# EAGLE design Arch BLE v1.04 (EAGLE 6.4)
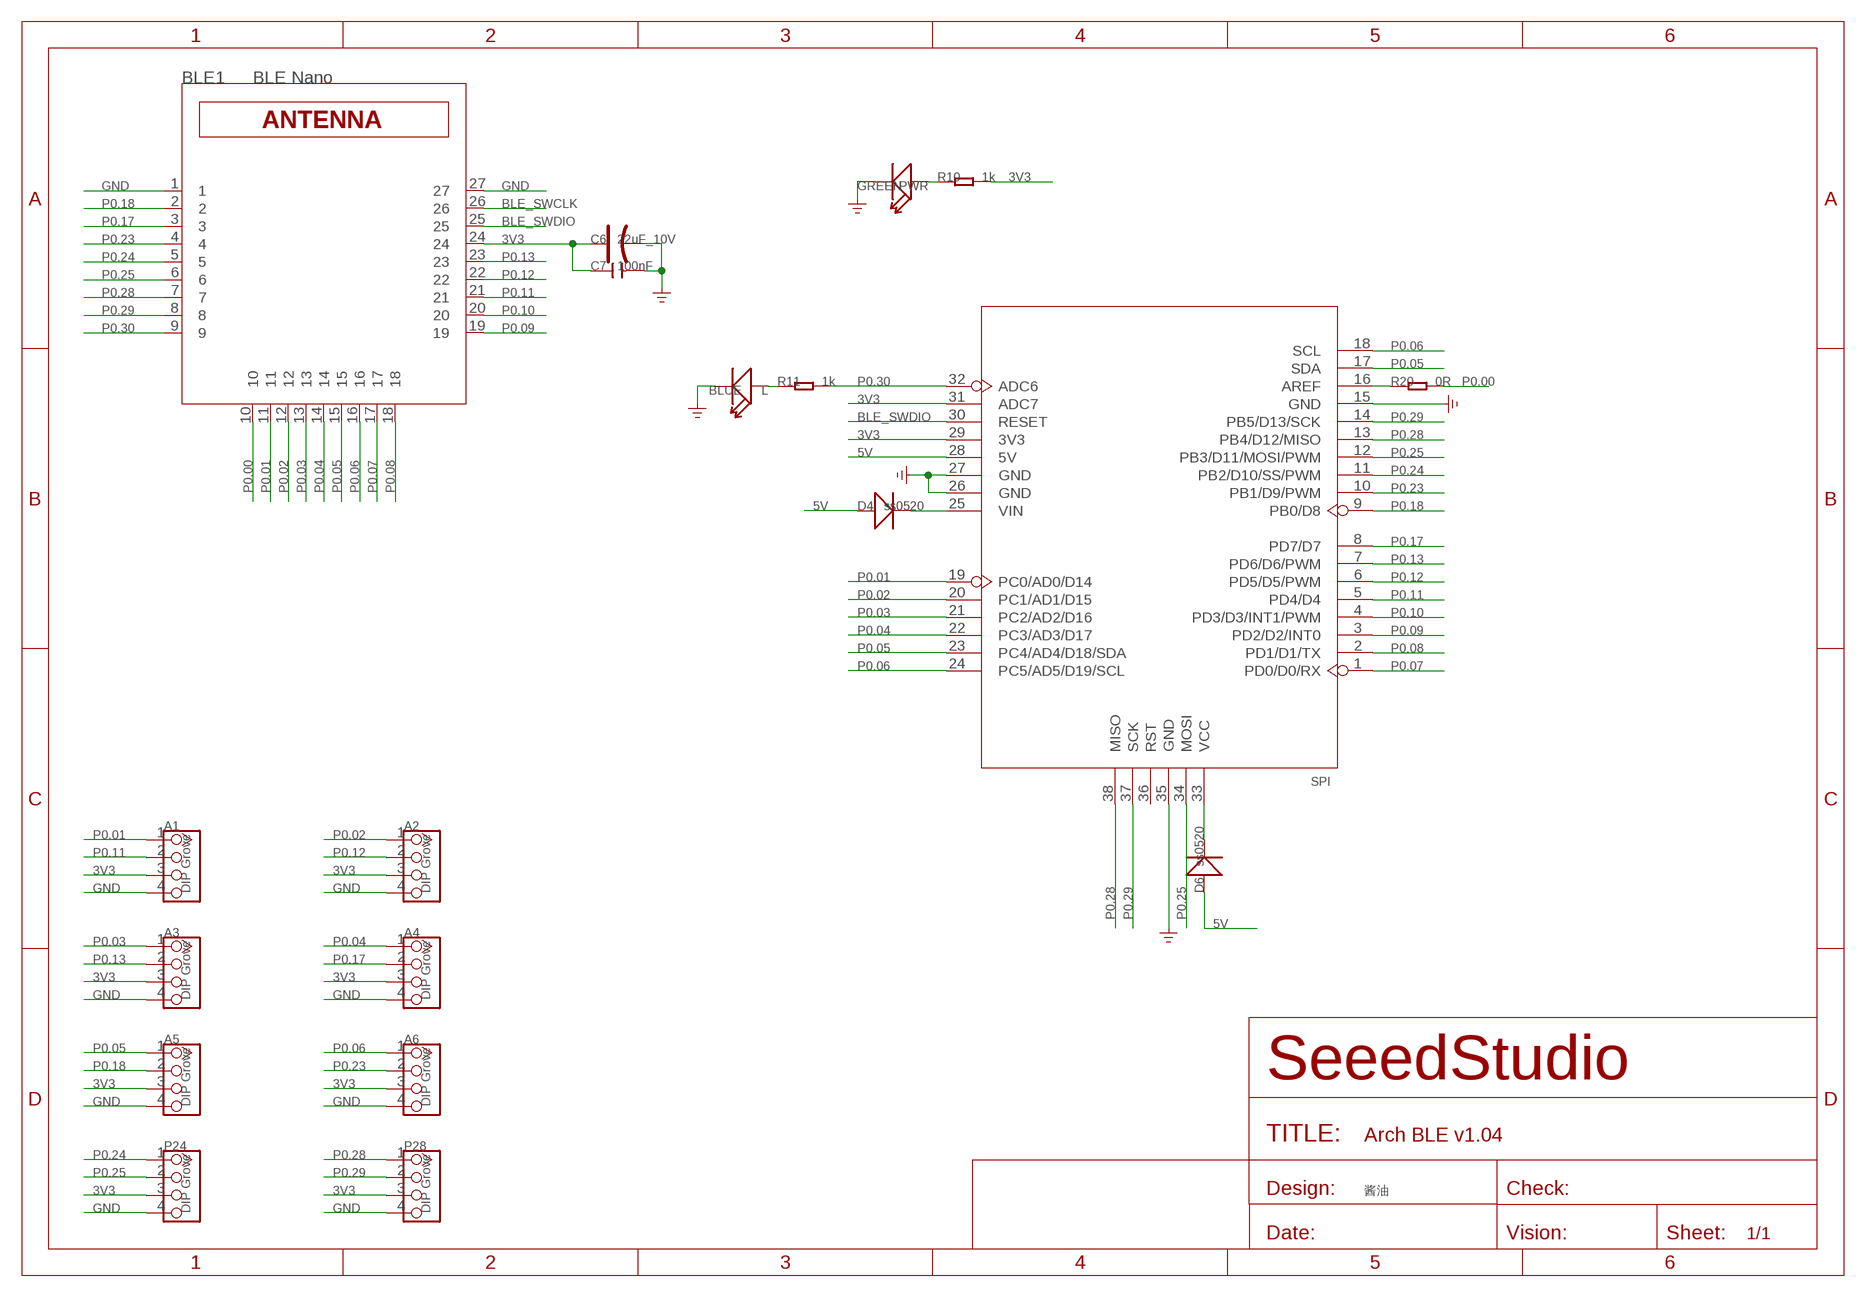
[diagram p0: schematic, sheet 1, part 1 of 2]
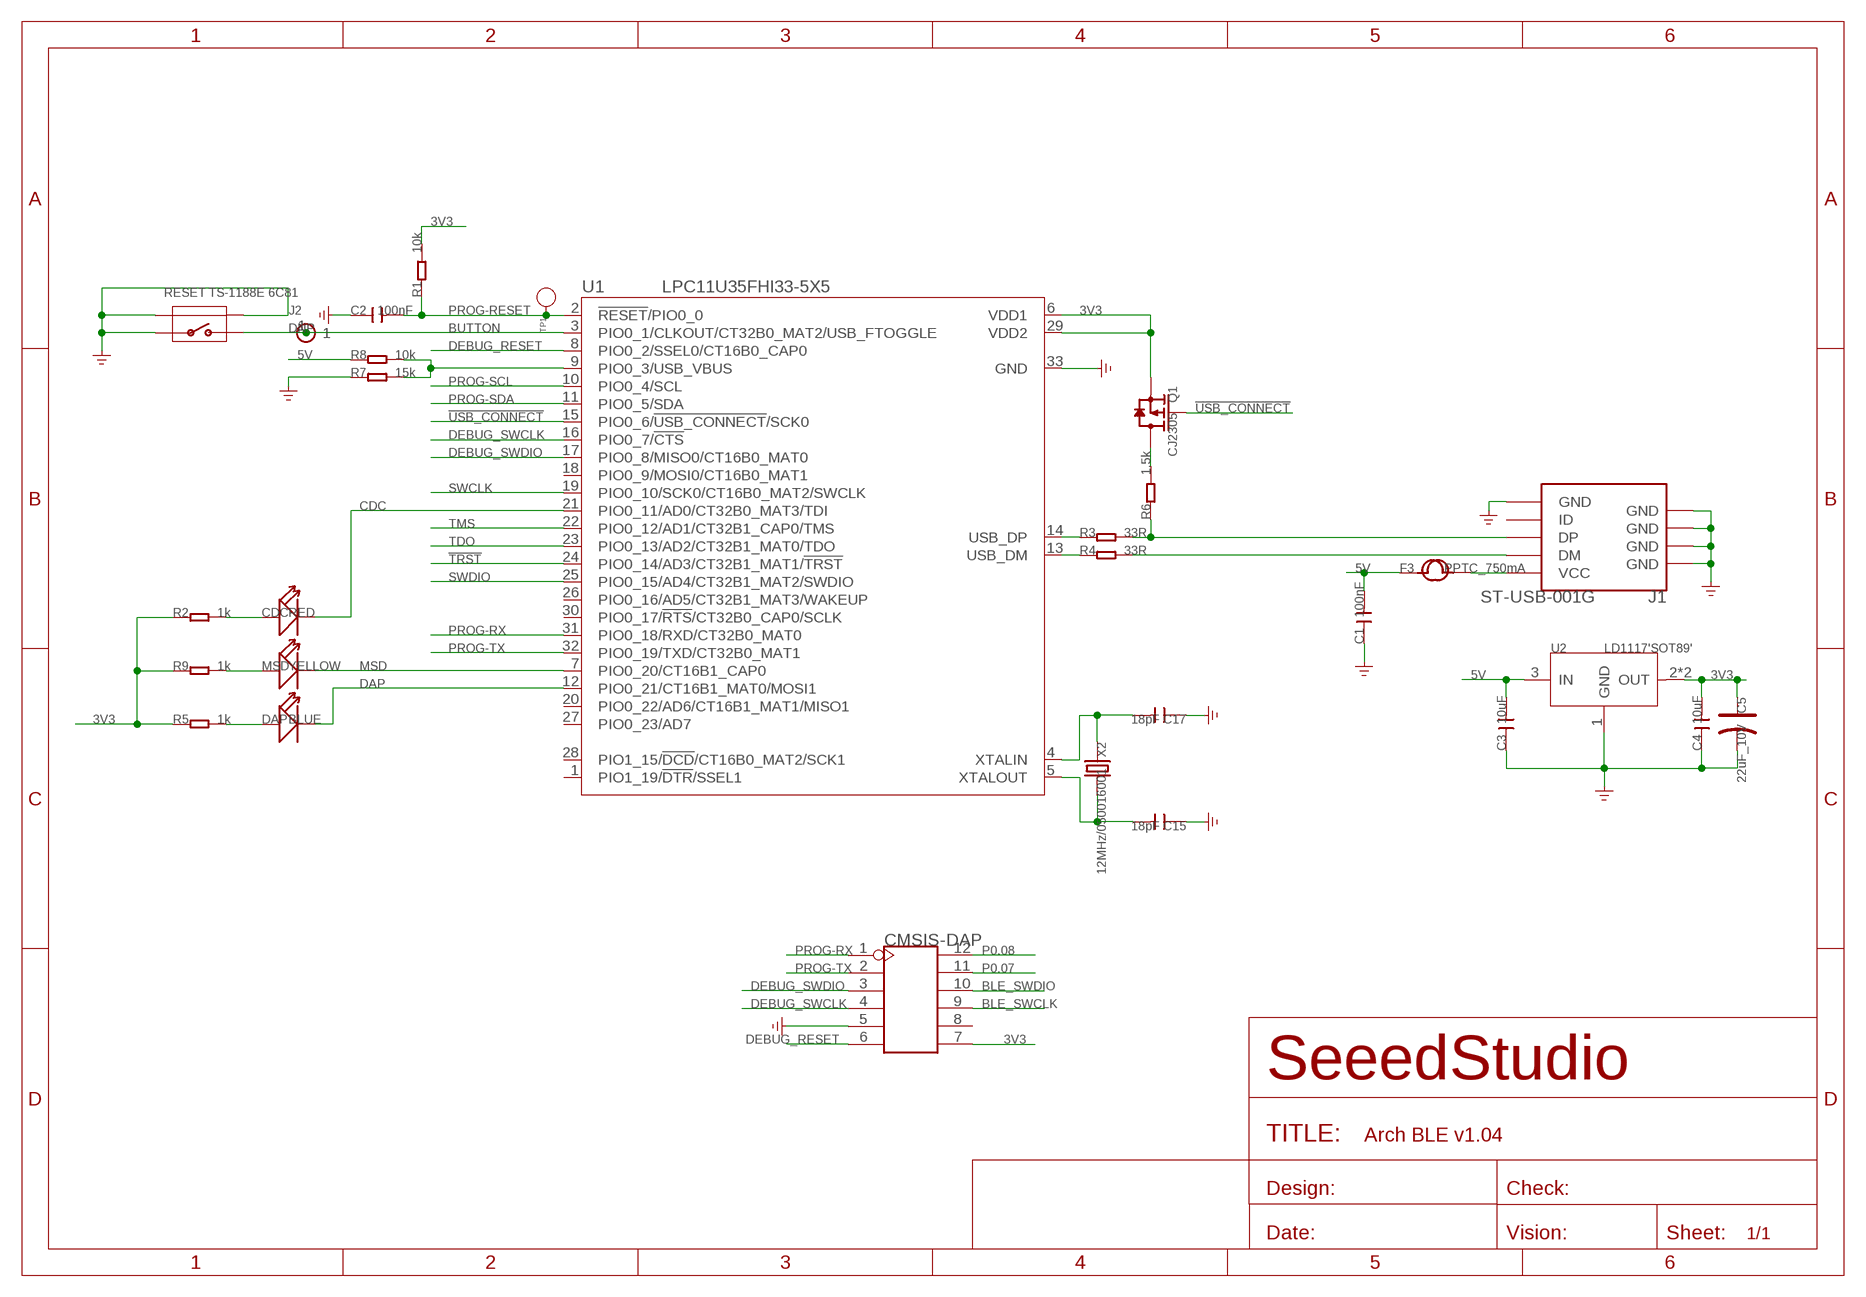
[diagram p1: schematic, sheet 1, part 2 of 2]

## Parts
A1  DIP Grove  TWIG-4P-2.0-2.0  [4P-2.0]
A2  DIP Grove  TWIG-4P-2.0-2.0  [4P-2.0]
A3  DIP Grove  TWIG-4P-2.0-2.0  [4P-2.0]
A4  DIP Grove  TWIG-4P-2.0-2.0  [4P-2.0]
A5  DIP Grove  TWIG-4P-2.0-2.0  [4P-2.0]
A6  DIP Grove  TWIG-4P-2.0-2.0  [4P-2.0]
BLE1  BLE Nano  SEEED_BLE_MODULE_001'PAD'  [SEEED_BLE_MODULE_PAD]
C1  100nF  C-0603  [C0603]
C2  100nF  C-0603  [C0603]
C3  10uF  C-0805  [C0805]
C4  10uF  C-0805  [C0805]
C5  22uF_10V  CAP-AVX-A  [AVX-A]
C6  22uF_10V  CAP-AVX-A  [AVX-A]
C7  100nF  C-0603  [C0603]
C15  18pF  C-0603  [C0603]
C17  18pF  C-0603  [C0603]
CDC  RED  LED'0603'  [LED-0603]
CMSIS-DAP  HEADER-2X6P-2.54  [2X6P-2.54]
D4  ss0520  D'1206'  [SOD123]
D6  ss0520  D'1206'  [SOD123]
DAP  BLUE  LED'0603'  [LED-0603]
F3  PPTC_750mA  FUSE'1206'  [F1206]
J1  ST-USB-001G  USB-MINIUSB-5P-MICRO  [MICRO-USB]
J2  DNP  HEADER-1P-35  [1P-65/35MIL]
L  BLUE  LED'0603'  [LED-0603]
MSD  YELLOW  LED'0603'  [LED-0603]
P24  DIP Grove  TWIG-4P-2.0-2.0  [4P-2.0]
P28  DIP Grove  TWIG-4P-2.0-2.0  [4P-2.0]
PWR  GREEN  LED'0603'  [LED-0603]
Q1  CJ2305  MOSFET-P'SI2323CDS/SI2305DS<BR>'  [SOT23]
R1  10k  R-0603  [R0603]
R2  1k  R-0603  [R0603]
R3  33R  R-0603  [R0603]
R4  33R  R-0603  [R0603]
R5  1k  R-0603  [R0603]
R6  1.5k  R-0603  [R0603]
R7  15k  R-0603  [R0603]
R8  10k  R-0603  [R0603]
R9  1k  R-0603  [R0603]
R10  1k  R-0603  [R0603]
R11  1k  R-0603  [R0603]
R20  0R  R-0603  [R0603]
RESET  TS-1188E 6C81  BUTTON-4P-REINFORCE'TS-1188E'  [4P-SMD-7X3.5X3.5H]
TP1  PAD-TEST-POINT'4545'  [TP_4545]
U1  LPC11U35FHI33-5X5  [HVQFN33]
U2  LD1117'SOT89'  [SOT89]
U5  ARDUINO-38P'WITH/O-SILK'  [ARDUINO-38P]
X2  12MHz/050016001  CRYSTAL'5032'  [2P-SMD-5X3.2]

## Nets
3V3: A1.3 A2.3 A3.3 A4.3 A5.3 A6.3 BLE1.24 C4.2 C5.+ C6.+ C7.1 CMSIS-DAP.7 P24.3 P28.3 Q1.2(S) R1.2 R2.1 R5.1 R9.1 R10.2 U1.6(VDD1) U1.29(VDD2) U2.2(OUT) U2.4(OUT) U5.29(3V3) U5.31(ADC7)
5V: C1.2 C3.2 D4.+ D6.+ F3.1 R8.1 U2.3(IN) U5.28(5V)
!TRST: U1.24(PIO0_14/AD3/CT32B1_MAT1/!TRST!)
!USB_CONNECT: Q1.1(G) U1.15(PIO0_6/!USB_CONNECT!/SCK0)
BLE_SWCLK: BLE1.26 CMSIS-DAP.9
BLE_SWDIO: BLE1.25 CMSIS-DAP.10 U5.30(RESET)
BUTTON: J2.1 RESET.2 U1.3(PIO0_1/CLKOUT/CT32B0_MAT2/USB_FTOGGLE)
CDC: CDC.- U1.21(PIO0_11/AD0/CT32B0_MAT3/TDI)
DAP: DAP.- U1.12(PIO0_21/CT16B1_MAT0/MOSI1)
DEBUG_RESET: CMSIS-DAP.6 U1.8(PIO0_2/SSEL0/CT16B0_CAP0)
DEBUG_SWCLK: CMSIS-DAP.4 U1.16(PIO0_7/!CTS!)
DEBUG_SWDIO: CMSIS-DAP.3 U1.17(PIO0_8/MISO0/CT16B0_MAT0)
GND: A1.4 A2.4 A3.4 A4.4 A5.4 A6.4 BLE1.1 BLE1.27 C1.1 C2.1 C3.1 C4.1 C5.- C6.- C7.2 C15.1 C17.1 CMSIS-DAP.5 J1.5(GND) J1.S1(GND) J1.S2(GND) J1.S3(GND) J1.S4(GND) J1.S5(GND) J1.S6(GND) L.- P24.4 P28.4 PWR.- R7.1 RESET.1 RESET.S1 RESET.S2 U1.33(GND) U2.1(GND) U5.15(GND) U5.26(GND) U5.27(GND) U5.35(GND)
MSD: MSD.- U1.7(PIO0_20/CT16B1_CAP0)
N$1: R3.1 U1.14(USB_DP)
N$2: PWR.+ R10.1
N$3: F3.2 J1.1(VCC)
N$4: CDC.+ R2.2
N$5: DAP.+ R5.2
N$6: MSD.+ R9.2
N$8: R20.1 U5.16(AREF)
N$11: L.+ R11.1
N$12: D4.- U5.25(VIN)
N$14: D6.- U5.33(VCC)
N$23: R4.1 U1.13(USB_DM)
N$32: J1.3(DP) R3.2 R6.1
N$34: C15.2 U1.5(XTALOUT) X2.2
N$37: C17.2 U1.4(XTALIN) X2.1
N$38: J1.2(DM) R4.2
N$39: Q1.3(D) R6.2
N$41: R7.2 R8.2 U1.9(PIO0_3/USB_VBUS)
P0.00: BLE1.10 R20.2
P0.01: A1.1 BLE1.11 U5.19(PC0/AD0/D14)
P0.02: A2.1 BLE1.12 U5.20(PC1/AD1/D15)
P0.03: A3.1 BLE1.13 U5.21(PC2/AD2/D16)
P0.04: A4.1 BLE1.14 U5.22(PC3/AD3/D17)
P0.05: A5.1 BLE1.15 U5.17(SDA) U5.23(PC4/AD4/D18/SDA)
P0.06: A6.1 BLE1.16 U5.18(SCL) U5.24(PC5/AD5/D19/SCL)
P0.07: BLE1.17 CMSIS-DAP.11 U5.1(PD0/D0/RX)
P0.08: BLE1.18 CMSIS-DAP.12 U5.2(PD1/D1/TX)
P0.09: BLE1.19 U5.3(PD2/D2/INT0)
P0.10: BLE1.20 U5.4(PD3/D3/INT1/PWM)
P0.11: A1.2 BLE1.21 U5.5(PD4/D4)
P0.12: A2.2 BLE1.22 U5.6(PD5/D5/PWM)
P0.13: A3.2 BLE1.23 U5.7(PD6/D6/PWM)
P0.17: A4.2 BLE1.3 U5.8(PD7/D7)
P0.18: A5.2 BLE1.2 U5.9(PB0/D8)
P0.23: A6.2 BLE1.4 U5.10(PB1/D9/PWM)
P0.24: BLE1.5 P24.1 U5.11(PB2/D10/SS/PWM)
P0.25: BLE1.6 P24.2 U5.12(PB3/D11/MOSI/PWM) U5.34(MOSI)
P0.28: BLE1.7 P28.1 U5.13(PB4/D12/MISO) U5.38(MISO)
P0.29: BLE1.8 P28.2 U5.14(PB5/D13/SCK) U5.37(SCK)
P0.30: BLE1.9 R11.2 U5.32(ADC6)
PROG-RESET: C2.2 R1.1 TP1.T U1.2(!RESET!/PIO0_0)
PROG-RX: CMSIS-DAP.1 U1.31(PIO0_18/RXD/CT32B0_MAT0)
PROG-SCL: U1.10(PIO0_4/SCL)
PROG-SDA: U1.11(PIO0_5/SDA)
PROG-TX: CMSIS-DAP.2 U1.32(PIO0_19/TXD/CT32B0_MAT1)
SWCLK: U1.19(PIO0_10/SCK0/CT16B0_MAT2/SWCLK)
SWDIO: U1.25(PIO0_15/AD4/CT32B1_MAT2/SWDIO)
TDO: U1.23(PIO0_13/AD2/CT32B1_MAT0/TDO)
TMS: U1.22(PIO0_12/AD1/CT32B1_CAP0/TMS)
Unconnected: CMSIS-DAP.8 J1.4(ID) U1.1(PIO1_19/!DTR!/SSEL1) U1.18(PIO0_9/MOSI0/CT16B0_MAT1) U1.20(PIO0_22/AD6/CT16B1_MAT1/MISO1) U1.26(PIO0_16/AD5/CT32B1_MAT3/WAKEUP) U1.27(PIO0_23/AD7) U1.28(PIO1_15/!DCD!/CT16B0_MAT2/SCK1) U1.30(PIO0_17/!RTS!/CT32B0_CAP0/SCLK) U5.36(RST)

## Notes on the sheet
- SPI
- 酱油

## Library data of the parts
A1-A6 P24 P28 = Connector:TWIG-4P-2.0
BLE1 = AMLib:SEEED_BLE_MODULE_001
C1-C4 C7 C15 C17 = Discrete:C*: Ceramic Capacitors
C5 C6 = Discrete:CAP*: Electrolytic Capacitors,Tantalum Capacitors and Super Capacitors
CDC DAP L MSD PWR = Discrete:LED*
CMSIS-DAP = Connector:HEADER-2X6P
D4 D6 = Discrete:D*
F3 = Discrete:FUSE
J1 = Connector :USB-MINIUSB-5P
J2 = Connector :HEADER-1P
Q1 = Discrete:MOSFET-P
R1-R11 R20 = Discrete:R*
RESET = Discrete:BUTTON-4P-REINFORCE: TS-1188E http://www.best-dz.com/?thread-374-2.html
TP1 = Discrete:PAD-TEST-POINT; PARTNO: DNP
U1 = AMLib:LPC11U35FHI33
U2 = IC:LD1117: Low Drop Fixed And Adjustable Positive Voltage Regulators http://www.datasheetcatalog.org/datasheet/SGSThomsonMicroelectronics/mXuqtqv.pdf
U5 = moudle:ARDUINO-38P
X2 = Discrete:CRYSTAL*: CRYSTAL

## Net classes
0 default: width 0.102 mm, drill 0.203 mm, clearance 0.102 mm

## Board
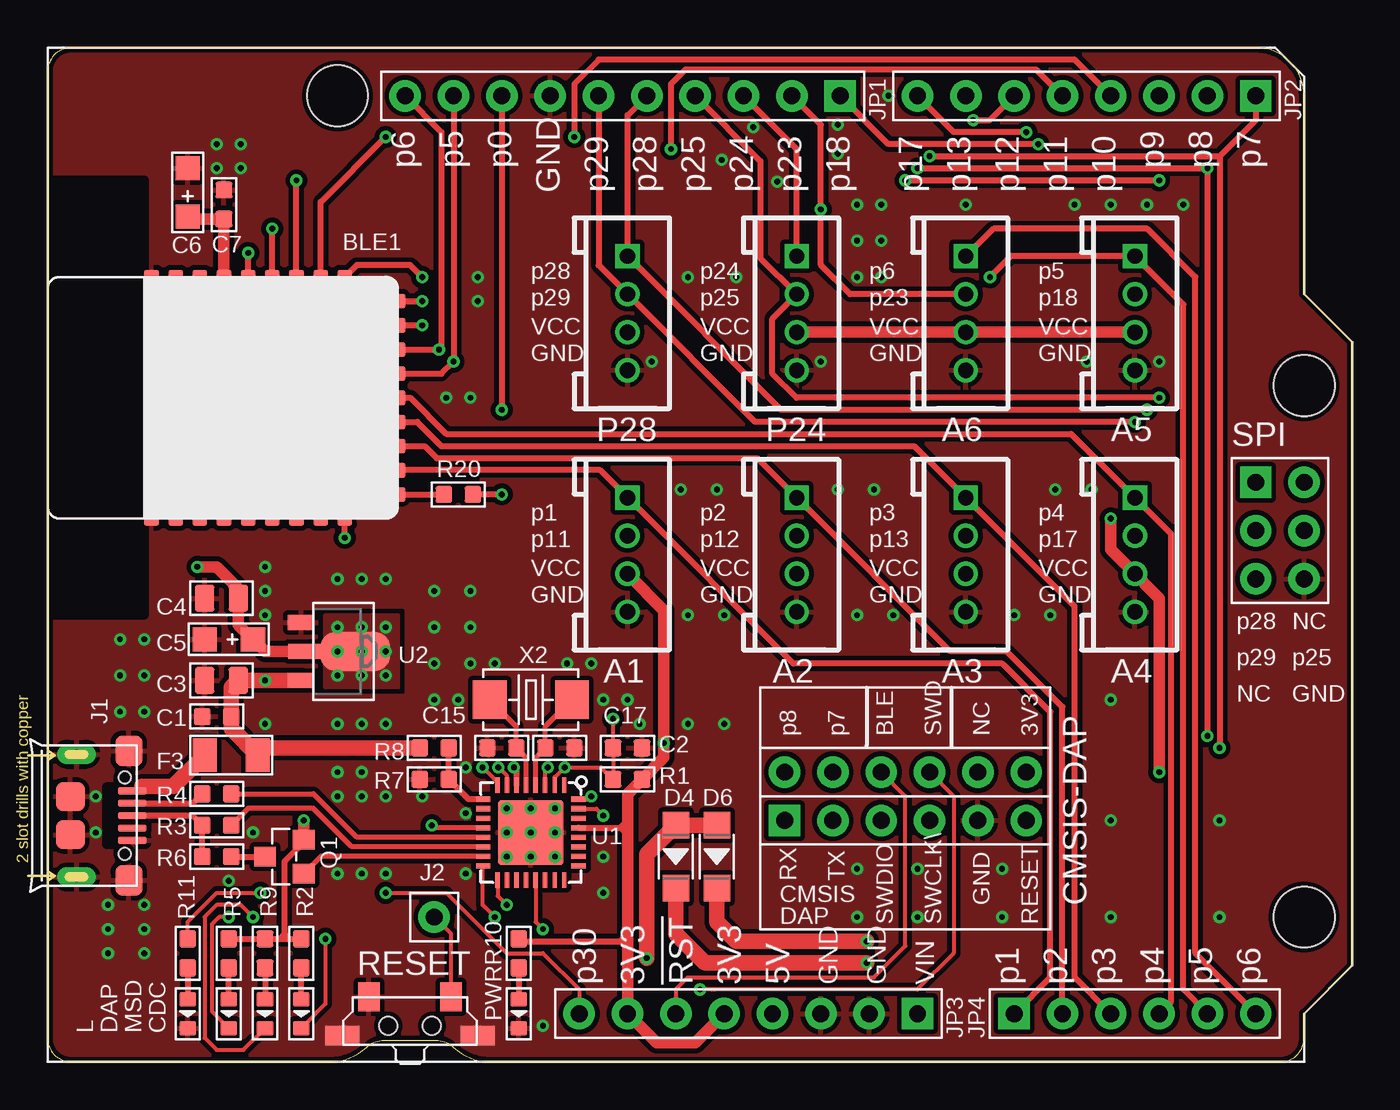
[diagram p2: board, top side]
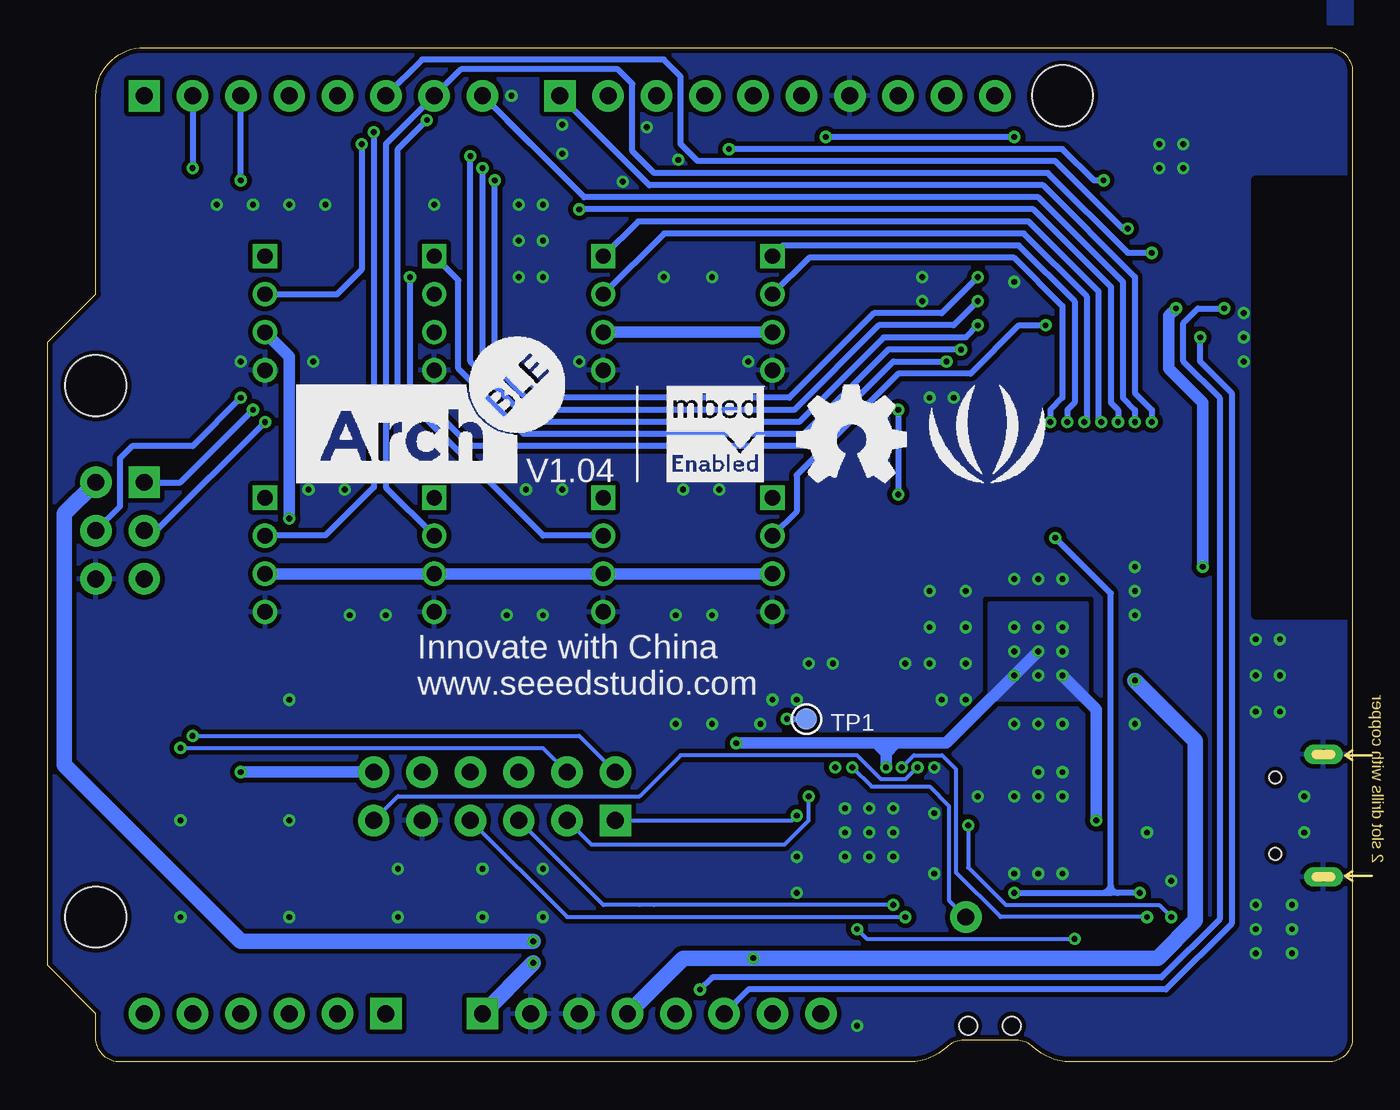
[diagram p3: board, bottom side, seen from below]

Size 68.58 x 53.34 mm. Coordinates in mm from the lower left corner, seen from the top.
Outline: 66.04,40.39 66.04,50.8 arc90 63.5,53.34 1.27,53.34 arc90 0,52.07 0,1.27 arc90 1.27,0 14.61,0 arc45 16.77,0.77 arc-45 17.67,1.14 20.43,1.14 arc-45 21.33,0.77 arc45 23.5,0 64.77,0 arc90 66.04,1.27 66.04,2.54 68.58,5.08 68.58,37.85 66.04,40.39
Copper layers (1*16): Top 0.035mm / dielectric 1.5mm / Bottom 0.035mm
Design rules "default *": minimum track width 6mil, minimum drill 12mil, track to track 6mil, track to pad 6mil, pad to pad 6mil, via to via 6mil, smd to smd 0mil, copper to edge 6mil, drill to drill 8mil, minimum pad ring 6mil, minimum via ring 6mil, stop-mask expansion 4mil, vias tented up to drill 25mil, thermal gap 10mil
tRestrict: area -0.6,23.5 to 5.1,46.4
bRestrict: area -0.6,23.5 to 5.1,46.4

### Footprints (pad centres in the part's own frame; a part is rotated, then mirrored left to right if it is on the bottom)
4P-2.0 = drill 0.8 pad 1.27 square: 1 -3,0 | drill 0.8 pad 1.27: 2 -1,0; 3 1,0; 4 3,0
SEEED_BLE_MODULE_PAD = smd 1.524 x 0.762: 1 -5.969,12.954; 2 -5.969,11.684; 3 -5.969,10.414; 4 -5.969,9.144; 5 -5.969,7.874; 6 -5.969,6.604; 7 -5.969,5.334; 8 -5.969,4.064; 9 -5.969,2.794; 19 5.969,2.794; 20 5.969,4.064; 21 5.969,5.334; 22 5.969,6.604; 23 5.969,7.874; 24 5.969,9.144; 25 5.969,10.414; 26 5.969,11.684; 27 5.969,12.954 | smd 0.762 x 1.524: 10 -5.08,0.381; 11 -3.81,0.381; 12 -2.54,0.381; 13 -1.27,0.381; 14 0,0.381; 15 1.27,0.381; 16 2.54,0.381; 17 3.81,0.381; 18 5.08,0.381
C0603 = smd 0.889 x 0.889: 1 -0.762,0; 2 0.762,0
C0805 = smd 1.016 x 1.397: 1 -0.889,0; 2 0.889,0
AVX-A = smd 1.27 x 1.27: + -1.27,0; - 1.27,0
LED-0603 = smd 0.762 x 0.889: + -0.762,0; - 0.762,0
2X6P-2.54 = drill 0.889 pad 1.651 square: 1 -1.27,6.35 | drill 0.889 pad 1.651: 2 -1.27,3.81; 3 -1.27,1.27; 4 -1.27,-1.27; 5 -1.27,-3.81; 6 -1.27,-6.35; 7 1.27,-6.35; 8 1.27,-3.81; 9 1.27,-1.27; 10 1.27,1.27; 11 1.27,3.81; 12 1.27,6.35
SOD123 = smd 1.397 x 1.397: + -1.651,0; - 1.651,0
F1206 = smd 1.27 x 1.778: 1 -1.397,0; 2 1.397,0
MICRO-USB = smd 0.381 x 1.524: 1 -1.3,-0.25; 2 -0.65,-0.25; 3 0,-0.25; 4 0.65,-0.25; 5 1.3,-0.25 | smd 1.6 x 1.397: S1 -3.4,-0.427; S6 3.4,-0.427 | drill 0.508 pad 1.016 long: S2 -3.226,-3.175; S5 3.226,-3.175 | smd 1.5 x 1.5: S3 -1,-3.5; S4 1,-3.5 | hole 0.635: -2,-0.65; 2,-0.65
1P-65/35MIL = drill 0.889 pad 1.651: 1 0,0
SOT23 = smd 1.016 x 1.143: 1 -0.889,-1.016; 2 0.889,-1.016; 3 0,1.016
R0603 = smd 0.889 x 0.889: 1 -0.762,0; 2 0.762,0
4P-SMD-7X3.5X3.5H = smd 1.143 x 1.524: 1 -2.159,1.524; 2 2.159,1.524 | smd 1.778 x 1.016: S1 -3.556,-0.508; S2 3.556,-0.508 | hole 0.95: -1.15,0; 1.15,0
TP_4545 = smd 1.143 x 1.143: T 0,0
HVQFN33 = smd 0.813 x 0.279: 1 -2.5,1.75; 2 -2.5,1.25; 3 -2.5,0.75; 4 -2.5,0.25; 5 -2.5,-0.25; 6 -2.5,-0.75; 7 -2.5,-1.25; 8 -2.5,-1.75; 17 2.5,-1.75; 18 2.5,-1.25; 19 2.5,-0.75; 20 2.5,-0.25; 21 2.5,0.25; 22 2.5,0.75; 23 2.5,1.25; 24 2.5,1.75 | smd 0.279 x 0.813: 9 -1.75,-2.5; 10 -1.25,-2.5; 11 -0.75,-2.5; 12 -0.25,-2.5; 13 0.25,-2.5; 14 0.75,-2.5; 15 1.25,-2.5; 16 1.75,-2.5; 25 1.75,2.5; 26 1.25,2.5; 27 0.75,2.5; 28 0.25,2.5; 29 -0.25,2.5; 30 -0.75,2.5; 31 -1.25,2.5; 32 -1.75,2.5 | smd 3.429 x 3.429: 33 0,0
SOT89 = smd 0.8 x 1.4: 1 -1.524,-1.905; 3 1.524,-1.905 | smd 0.8 x 1.9: 2 0,-1.651 | smd 2.032 x 3.65: 4 0,0.94
ARDUINO-38P = drill 0.889 pad 1.651 square: 1 63.5,50.8; 9 41.656,50.8; 19 50.8,2.54; 25 45.72,2.54; 38 63.5,30.48 | drill 0.889 pad 1.651: 2 60.96,50.8; 3 58.42,50.8; 4 55.88,50.8; 5 53.34,50.8; 6 50.8,50.8; 7 48.26,50.8; 8 45.72,50.8; 10 39.116,50.8; 11 36.576,50.8; 12 34.036,50.8; 13 31.496,50.8; 14 28.956,50.8; 15 26.416,50.8; 16 23.876,50.8; 17 21.336,50.8; 18 18.796,50.8; 20 53.34,2.54; 21 55.88,2.54; 22 58.42,2.54; 23 60.96,2.54; 24 63.5,2.54; 26 43.18,2.54; 27 40.64,2.54; 28 38.1,2.54; 29 35.56,2.54; 30 33.02,2.54; 31 30.48,2.54; 32 27.94,2.54; 33 66.04,30.48; 34 66.04,27.94; 35 66.04,25.4; 36 63.5,25.4; 37 63.5,27.94 | hole 3.2: 15.24,50.8; 66.04,35.56; 66.04,7.62
2P-SMD-5X3.2 = smd 1.778 x 2.032: 1 -2.159,0; 2 2.159,0

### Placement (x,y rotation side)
A1  30.48,26.67 270 top
A2  39.37,26.67 270 top
A3  48.26,26.67 270 top
A4  57.15,26.67 270 top
A5  57.15,39.37 270 top
A6  48.26,39.37 270 top
BLE1  18.41,34.93 90 top
C1  8.89,18.16 0 top
C2  30.48,16.51 180 top
C3  9.14,20.07 0 top
C4  9.14,24.39 0 top
C5  9.53,22.23 180 top
C6  7.37,45.72 90 top
C7  9.27,45.09 90 top
C15  23.88,16.51 0 top
C17  26.92,16.51 180 top
CDC  13.34,2.54 270 top
CMSIS-DAP  45.09,13.97 90 top
D4  33.02,10.8 270 top
D6  35.18,10.8 270 top
DAP  9.53,2.54 270 top
F3  9.65,16.13 180 top
J1  4.7,12.96 270 top
J2  20.32,7.62 0 top
L  7.37,2.54 270 top
MSD  11.43,2.54 270 top
P24  39.37,39.37 270 top
P28  30.48,39.37 270 top
PWR  24.77,2.54 270 top
Q1  12.45,10.8 90 top
R1  30.48,14.86 0 top
R2  13.34,5.72 270 top
R3  8.89,12.45 180 top
R4  8.89,14.1 180 top
R5  9.53,5.72 270 top
R6  8.89,10.8 0 top
R7  20.32,14.86 0 top
R8  20.32,16.51 0 top
R9  11.43,5.72 270 top
R10  24.77,5.72 90 top
R11  7.37,5.72 90 top
R20  21.59,29.85 180 top
RESET  19.05,1.91 0 top
TP1  28.7,18.04 0 bottom
U1  25.4,12.07 270 top
U2  15.24,21.59 270 top
U5  0,0 0 top
U$5  [SEEED_MASK]  3.81,49.53 0 top
X2  25.4,19.05 180 top

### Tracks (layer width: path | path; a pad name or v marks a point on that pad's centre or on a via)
3V3  (via drill 0.3 pad 0.64)
  Top 0.305: U1.6 24.65,15.36 v24.51,15.5 | Q1.2 13.59,11.69 12.45,10.54 12.45,6.73 | R5.1 R9.1 12.19,6.48 | 12.19,6.48 12.45,6.48 | 12.45,6.48 12.7,6.48 | 12.7,6.48 R2.1 | 12.45,6.73 12.45,6.48 | 12.19,6.48 12.45,6.73 | 12.45,6.73 12.7,6.48 | U1.29 30.09,12.32 | 30.1,12.32 30.36,12.32 30.48,12.19 | R10.2 24.77,6.35 30.1,6.35 | 30.1,6.35 30.48,6.35 | 30.09,12.32 30.35,12.57 | 30.09,12.32 30.1,12.32 | 30.1,12.32 30.48,11.94 | 30.1,6.35 30.48,6.73 | 30.1,6.35 30.48,5.97
  Top 0.61: U2.4 U2.2 11.43,21.59 C5.+ 10.03,22.99 C4.2 10.03,24.89 8.89,26.04 v7.87,26.04 | Q1.2 v13.46,12.7 | A1.3 30.48,25.66 32.38,23.75 v32.38,16.77 32.38,16 R1.2 | R1.2 31.37,14.86 | U5.29 34.04,1.02 32,1.02 U5.31 30.48,5.97 30.48,6.35 30.48,6.73 30.48,11.94 30.48,12.19 30.48,14.1 R1.2 | C6.+ 7.49,44.32 C7.1 BLE1.24 v9.27,39.63 | A5.3 A6.3 P24.3 | v55.88,28.58 55.88,26.94 56.81,26.01 | 56.81,26.01 A4.3 | 56.81,26.01 56.81,25.99 58.42,24.39 v58.42,15.24
  Bottom 0.61: v13.46,12.7 13.46,18.54 v15.24,20.32 | v16.51,21.59 21.34,16.77 24,16.77 | v7.87,26.04 7.87,34.67 9.65,36.45 9.65,39.24 v9.27,39.63 | A4.3 A3.3 A2.3 A1.3 | P28.3 P24.3 | 24,16.77 24.51,16.77 | 24.51,16.77 25.02,16.77 | 25.02,16.77 v32.38,16.77 | v24.51,15.5 24.51,16.26 | 24.51,16.26 24.51,16.77 | 24,16.77 24.51,16.26 | 24.51,16.26 25.02,16.77 | A5.3 57.15,38.36 55.88,37.09 v55.88,28.58 | v58.42,15.24 CMSIS-DAP.7
  other vias: 15.24,22.86 16.51,22.86 17.78,22.86 17.78,21.59 15.24,21.59 16.51,20.32 17.78,20.32
  pour Top (isolate 0.254, no thermals): 14.61,23.5 18.41,23.5 18.41,19.69 14.61,19.69
  pour Bottom: 19.05,24.13 13.97,24.13 13.97,19.05 19.05,19.05
5V  (via drill 0.3 pad 0.64)
  Top 0.813: U2.3 v11.43,20.07 C3.2 9.65,19.69 C1.2 9.65,17.53 F3.1 11.43,16.51 R8.1 | v31.5,5.46 31.5,10.92 D4.+ D6.+
  Bottom 0.813: v11.43,20.07 8.26,16.89 8.26,7.45 10.24,5.46 v31.5,5.46 35.18,5.46 U5.28
!USB_CONNECT
  Top 0.254: U1.15 14.37,10.82 Q1.1
BLE_SWCLK  (via drill 0.3 pad 0.64)
  Top 0.203: CMSIS-DAP.9 47.62,13.97 47.62,5.72 45.72,3.81 35.05,3.81 34.92,3.81 v34.29,3.81
  Top 0.305: BLE1.26 v6.73,39.63
  Bottom 0.305: v6.73,39.63 8.13,39.63 8.89,38.86 8.89,36.83 6.99,34.93 6.99,7.51 10.04,4.45 33.66,4.45 v34.29,3.81
BLE_SWDIO  (via drill 0.3 pad 0.64)
  Top 0.203: CMSIS-DAP.10 45.09,13.97 45.09,6.1 43.43,4.45 33.66,4.45 33.02,3.81 U5.30
  Top 0.305: BLE1.25 v8,38.1
  Bottom 0.305: U5.30 31.75,3.81 9.8,3.81 6.35,7.27 6.35,35.18 8,36.83 v8,38.1
BUTTON  (via drill 0.3 pad 0.64)
  Top 0.203: U1.3 26.15,15.36 v26.29,15.5 | RESET.2 21.21,6.73 J2.1
  Bottom 0.203: v26.29,15.5 25.27,14.48 22.23,14.48 21.21,13.46 21.21,8.51 J2.1
CDC  (via drill 0.3 pad 0.64)
  Top 0.203: v26.04,6.99 25.65,7.37 U1.21 | v14.61,6.48 14.61,3.05 CDC.-
  Bottom 0.203: v26.04,6.99 25.53,6.48 v14.61,6.48
DAP  (via drill 0.3 pad 0.64)
  Top 0.203: v9.53,7.62 9.02,7.62 8.64,7.24 8.64,2.67 DAP.-
  Top 0.254: U1.12 20.32,12.32 v20.19,12.45
  Bottom 0.203: v20.19,12.45 20.19,10.23 18.22,8.26 10.16,8.26 v9.53,7.62
DEBUG_RESET  (via drill 0.3 pad 0.64)
  Top 0.203: 23.65,14.71 v22.86,15.5
  Top 0.254: U1.8 23.65,14.71
  Bottom 0.203: v22.86,15.5 23.5,14.86 24.77,14.86 26.04,16.13 35.31,16.13 37.47,13.97 50.16,13.97 CMSIS-DAP.6
DEBUG_SWCLK  (via drill 0.3 pad 0.64)
  Top 0.203: 22.76,10.32 22.73,10.29 22.87,10.29 U1.16 22.86,10.28 22.86,8.26 v23.5,7.62
  Bottom 0.203: v23.5,7.62 41.27,7.62 CMSIS-DAP.4
DEBUG_SWDIO  (via drill 0.3 pad 0.64)
  Top 0.203: 23.62,9.54 U1.17 23.65,8.74 v24.13,8.26
  Bottom 0.203: v24.13,8.26 36.7,8.26 37.47,8.26 39.37,8.26 CMSIS-DAP.3
GND  (via drill 0.3 pad 0.64)
  other vias: 26.04,1.91 19.68,13.97 17.78,13.97 16.51,15.24 16.51,13.97 15.24,17.78 16.51,17.78 17.78,17.78 15.24,15.24 15.24,13.97 21.59,19.05 20.32,19.05 29.21,19.05 30.48,19.05 31.11,17.78 21.97,13.08 21.97,9.91 15.24,9.91 16.51,9.91 17.78,9.91 28.57,20.96 27.3,20.96 22.23,20.96 23.5,20.96 10.79,12.07 9.53,9.53 11.43,17.78 3.17,6.99 5.08,8.26 3.17,8.26 5.08,6.99 5.08,22.23 5.08,20.32 5.08,18.42 3.81,18.42 3.81,20.32 3.81,22.23 11.43,23.5 11.43,24.77 8.89,48.26 8.89,46.99 10.16,46.99 10.16,48.26 20.32,20.96 20.32,22.86 20.32,24.77 22.23,24.77 22.23,22.86 15.24,25.4 16.51,25.4 17.78,25.4 11.43,26.04 36.2,41.28 33.66,41.28 59.69,45.09 57.78,45.09 55.88,45.09 53.98,45.09 48.26,45.09 43.81,45.09 42.55,45.09 42.55,43.18 43.81,43.18 43.81,41.28 42.55,41.28 17.78,41.02 38.35,46.29 44.2,50.8 41.53,49.28 41.53,47.75 37.08,49.15 35.43,47.44 5.71,36.83 5.71,39.37 5.71,38.1 22.61,41.28 22.61,40.01 22.23,34.93 20.95,34.93 3.17,5.72 5.08,5.72 2.54,13.97 2.54,12.07 24.13,13.34 25.4,13.34 26.67,13.34 26.67,12.07 25.4,12.07 24.13,12.07 24.13,10.8 25.4,10.8 26.67,10.8 33.66,23.5 35.56,23.5 42.55,23.5 44.45,23.5 50.8,23.5 52.7,23.5 33.27,30.1 35.18,30.1 41.53,30.1 52.96,30.1 40.64,36.83 31.75,36.83 54.61,36.83 58.42,36.83 43.43,30.1 54.86,30.1 21.97,15.5 29.21,8.89 29.21,10.8 61.59,12.7 61.59,7.62 45.72,10.16 45.72,7.62 50.16,10.16 50.16,7.62 42.55,10.16 42.55,7.62 55.88,19.05 55.88,12.7 55.88,7.62 35.56,17.78 33.66,17.78
  pour Bottom: 0,55.88 1.27,55.88 1.27,54.61 0,54.61
  pour Bottom (isolate 0.254, rank 6): 0,53.34 68.58,53.34 68.58,0 0,0
  pour Top (isolate 0.254, rank 6): 0,53.34 68.58,53.34 68.58,0 0,0
MSD  (via drill 0.3 pad 0.64)
  Top 0.203: U1.7 24.15,15.03 v23.69,15.5 | v10.79,7.62 10.16,8.26 8.89,8.26 8.26,7.62 8.26,1.27 8.89,0.64 10.29,0.64 MSD.-
  Bottom 0.203: v23.69,15.5 23.05,16.13 21.57,16.13 20.83,15.39 20.83,9.96 18.49,7.62 v10.79,7.62
N$1
  Top 0.254: U1.14 15.99,11.32 13.97,13.34 10.54,13.34 R3.1
N$2
  Top 0.305: R10.1 PWR.+
N$3
  Top 0.203: J1.1 4.95,14.26 5.05,14.26 5.08,14.23
  Top 0.305: 4.95,14.48 4.95,14.26
  Top 0.813: 4.95,14.48 6.6,14.48 F3.2
N$4
  Top 0.305: CDC.+ R2.2
N$5
  Top 0.305: DAP.+ R5.2
N$6
  Top 0.305: R9.2 MSD.+
N$8  (via drill 0.3 pad 0.64)
  Top 0.305: U5.16 v23.88,34.29 | v23.88,29.85 R20.1
  Bottom 0.305: v23.88,34.29 v23.88,29.85
N$11
  Top 0.305: R11.1 L.+
N$12  (via drill 0.3 pad 0.64)
  Top 0.813: D4.- 33.02,6.73 34.54,5.21 v43.05,5.21
  Bottom 0.813: v43.05,5.21 U5.25
N$14  (via drill 0.3 pad 0.64)
  Top 0.813: D6.- 35.18,7.37 36.2,6.35 v43.05,6.35
  Bottom 0.813: v43.05,6.35 58.42,6.35 67.69,15.62 67.69,28.83 U5.33
N$23
  Top 0.254: U1.13 16.25,11.82 13.97,14.1 R4.1
N$32
  Top 0.305: J1.3 7.62,12.96 R3.2 R6.1
N$34
  Top 0.254: U1.5 25.15,16 C15.2 24.64,17.65 X2.2
N$37
  Top 0.254: U1.4 25.65,16 C17.2 26.16,17.65 X2.1
N$38
  Top 0.305: J1.2 7.63,13.61 R4.2
N$39
  Top 0.305: R6.2 Q1.3
N$41
  Top 0.305: U1.9 22.13,13.82 R7.2 R8.2
P0.00
  Top 0.305: BLE1.10 R20.2
P0.01
  Top 0.305: U5.19 52.7,4.45 52.7,18.42 50.16,20.96 39.2,20.96 A1.1 29.04,31.12 BLE1.11
P0.02
  Top 0.305: U5.20 53.34,18.67 50.42,21.59 47.45,21.59 A2.1 37.29,31.75 20.45,31.75 19.81,32.39 BLE1.12
P0.03
  Top 0.305: U5.21 53.98,4.45 53.98,23.96 A3.1 45.55,32.39 20.7,32.39 19.43,33.66 BLE1.13
P0.04
  Top 0.305: U5.22 59.05,3.18 59.05,27.77 A4.1 53.8,33.02 20.95,33.02 19.05,34.93 BLE1.14
P0.05  (via drill 0.3 pad 0.64)
  Top 0.305: U5.17 v21.34,36.83 20.7,36.2 BLE1.15 | U5.23 59.69,3.81 59.69,39.83 A5.1 50.62,42.37 v49.53,41.28
  Bottom 0.305: v21.34,36.83 24.13,36.83 28.57,32.39 46.35,32.39 49.53,35.56 v49.53,41.28
P0.06  (via drill 0.3 pad 0.64)
  Top 0.305: A6.1 49.7,43.82 57.78,43.82 60.33,41.28 60.33,5.72 U5.24 | U5.18 20.7,48.9 20.7,37.59 v20.57,37.47 BLE1.16
  Bottom 0.305: v20.57,37.47 24.38,37.47 28.83,33.02 43.56,33.02 46.99,36.45 46.99,41.1 A6.1
P0.07  (via drill 0.3 pad 0.64)
  Top 0.305: BLE1.17 v19.68,38.74 | v46.35,47.63 61.59,47.63 | U5.1 63.5,49.53 61.59,47.63 | 61.59,47.63 v61.59,16.51
  Bottom 0.203: v61.59,16.51 42.55,16.51 CMSIS-DAP.11
  Bottom 0.305: v19.68,38.74 20.32,38.1 24.64,38.1 29.08,33.66 43.18,33.66 46.35,36.83 v46.35,47.63
P0.08  (via drill 0.3 pad 0.64)
  Top 0.305: v45.72,46.99 v60.96,46.99 v60.96,17.15 | BLE1.18 v19.68,40.01
  Bottom 0.203: v60.96,17.15 40.64,17.15 CMSIS-DAP.12
  Bottom 0.305: v19.68,40.01 20.95,38.74 24.89,38.74 29.34,34.29 42.8,34.29 45.72,37.21 v45.72,46.99 | U5.2 v60.96,46.99
P0.09  (via drill 0.3 pad 0.64)
  Top 0.305: v19.68,41.28 19.05,41.91 16.26,41.91 15.62,41.28 BLE1.19 | v45.09,46.36 v58.42,46.36
  Bottom 0.305: v19.68,41.28 21.59,39.37 25.15,39.37 29.59,34.93 42.42,34.93 45.09,37.59 v45.09,46.36 | v58.42,46.36 U5.3
P0.10  (via drill 0.3 pad 0.64)
  Top 0.305: U5.4 53.98,52.71 28.96,52.71 27.69,51.44 v27.69,48.64 | v17.78,48.64 14.35,45.21 BLE1.20
  Bottom 0.305: v27.69,48.64 v17.78,48.64
P0.11  (via drill 0.3 pad 0.64)
  Top 0.305: U5.5 51.94,52.2 33.53,52.2 32.77,51.44 v32.77,48.01 | v13.08,46.36 BLE1.21 13.08,39.75 14.1,38.74 v16.13,38.74
  Bottom 0.305: v32.77,48.01 15.24,48.01 13.59,46.36 v13.08,46.36 | A1.2 29.21,28.94 29.21,30.86 23.88,36.2 20.07,36.2 17.53,38.74 v16.13,38.74
P0.12  (via drill 0.3 pad 0.64)
  Top 0.305: v48.64,49.53 49.53,49.53 U5.6 | BLE1.22 v11.81,43.82
  Bottom 0.305: U5.6 48.9,52.71 36.2,52.71 35.31,51.82 35.31,48.26 34.42,47.37 15.62,47.37 12.06,43.82 v11.81,43.82 | A2.2 42.53,27.67 50.16,35.31 50.16,48.01 v48.64,49.53
P0.13  (via drill 0.3 pad 0.64)
  Top 0.305: BLE1.23 v10.54,42.55
  Bottom 0.305: A3.2 50.8,30.21 50.8,48.26 U5.7 46.86,52.2 38.61,52.2 37.85,51.44 37.85,47.88 36.7,46.74 16,46.74 11.81,42.55 v10.54,42.55
P0.17  (via drill 0.3 pad 0.64)
  Top 0.305: v51.44,48.9 47.62,48.9 U5.8 | v11.43,33.66 11.43,33.28 8,29.85 BLE1.3
  Bottom 0.305: 43.18,48.26 U5.8 40.39,45.47 16.51,45.47 12.06,41.02 12.06,34.93 11.43,34.29 v11.43,33.66 | v51.44,48.9 51.44,30.23 53.98,27.69 57.13,27.69 A4.2
P0.18  (via drill 0.3 pad 0.64)
  Top 0.305: v52.07,48.26 44.2,48.26 U5.9 | v10.54,33.66 6.73,29.85 BLE1.2
  Bottom 0.305: U5.9 36.96,46.1 16.26,46.1 11.43,41.28 11.43,35.18 10.54,34.29 v10.54,33.66 | v52.07,48.26 52.07,41.66 53.36,40.37 A5.2
P0.23  (via drill 0.3 pad 0.64)
  Top 0.305: U5.10 40.64,49.28 v40.64,44.83 40.64,41.91 42.18,40.37 A6.2 | v12.32,33.66 12.32,32.89 9.27,29.85 BLE1.4
  Bottom 0.305: v40.64,44.83 16.76,44.83 12.7,40.77 12.7,34.67 12.32,34.29 v12.32,33.66
P0.24  (via drill 0.3 pad 0.64)
  Top 0.305: P24.1 39.37,48.01 U5.11 | v13.21,33.66 13.21,32.51 10.54,29.85 BLE1.5
  Bottom 0.305: P24.1 37.54,44.2 17.02,44.2 13.34,40.51 13.34,33.78 v13.21,33.66
P0.25  (via drill 0.3 pad 0.64)
  Top 0.305: U5.12 37.47,47.37 37.47,42.28 P24.2 38.1,39.1 38.1,36.2 39.37,34.93 v58.42,34.93 | v14.1,33.66 14.1,32.13 11.81,29.85 BLE1.6
  Bottom 0.305: P24.2 36.18,43.56 17.27,43.56 13.97,40.26 13.97,33.78 v14.1,33.66 | U5.34 64.77,29.21 64.77,31.75 64.14,32.39 60.96,32.39 v58.42,34.93
P0.28  (via drill 0.3 pad 0.64)
  Top 0.305: U5.13 30.48,49.79 P28.1 38.56,34.29 v57.78,34.29 | v14.99,33.66 14.99,31.75 13.08,29.85 BLE1.7
  Bottom 0.305: P28.1 29.92,42.93 17.53,42.93 14.61,40.01 14.61,34.67 14.99,34.29 v14.99,33.66 | U5.38 61.59,30.48 v57.78,34.29
P0.29  (via drill 0.3 pad 0.64)
  Top 0.305: U5.14 28.96,41.9 P28.2 37.2,33.66 v57.15,33.66 | v15.88,33.66 15.88,31.37 14.35,29.85 BLE1.8
  Bottom 0.305: P28.2 28.56,42.29 17.78,42.29 15.24,39.75 15.24,34.93 15.88,34.29 v15.88,33.66 | U5.37 62.87,27.94 v57.15,33.66
P0.30  (via drill 0.3 pad 0.64)
  Top 0.203: v17.78,8.89 20.95,8.89 24.13,5.72 26.04,5.72 27.94,3.81 U5.32 | R11.2 7.37,7.37 8.89,8.89 v11.18,8.89
  Top 0.305: v15.62,27.56 BLE1.9
  Bottom 0.305: 12.7,8.89 12.7,9.27 | 12.7,9.27 12.7,24.64 v15.62,27.56 | v11.18,8.89 12.32,8.89 | 12.32,8.89 12.7,8.89 | v17.78,8.89 13.08,8.89 | 13.08,8.89 12.7,8.89 | 12.7,9.27 arc60 13.08,8.89 | 12.7,9.27 arc-90 12.32,8.89
PROG-RESET  (via drill 0.3 pad 0.64)
  Top 0.203: U1.2 26.65,14.97 v27.18,15.5 29.08,15.5 R1.1 C2.2 v29.72,18.04
  Bottom 0.305: v29.72,18.04 TP1.T
PROG-RX  (via drill 0.3 pad 0.64)
  Top 0.203: U1.31 28.85,13.32 v29.21,12.96
  Bottom 0.203: CMSIS-DAP.1 29.46,12.7 v29.21,12.96
PROG-TX  (via drill 0.3 pad 0.64)
  Top 0.203: U1.32 28.42,13.82 v28.57,13.97
  Bottom 0.203: CMSIS-DAP.2 40.01,11.43 29.84,11.43 28.57,12.7 v28.57,13.97

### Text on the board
tPlace: JP1 | JP2 | p6 | p5 | p0 | p9 | p8 | p7 | GND | p29 | p28 | p25 | p24 | p23 | p18 | p17 | p13 | p12 | p11 | p10 | p28 | p24 | p6 | p5 | p29 | p25 | p23 | p18 | VCC | VCC | VCC | VCC | GND | GND | GND | GND | SPI | p1 | p2 | p3 | p4 | p11 | p12 | p13 | p17 | VCC | VCC | VCC | VCC | GND | GND | GND | GND | p28 | NC | p29 | p25 | NC | GND | p8 | p7 | BLE | SWD | NC | 3V3 | RX | TX | CMSIS | GND | DAP | SWDIO | SWCLK\ | RESET | p30 | 3V3 | !RST | 3V3 | 5V | GND | GND | VIN | p1 | p2 | p3 | p4 | p5 | p6 | JP3 | JP4
bPlace: V1.04 | Innovate with China | www.seeedstudio.com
